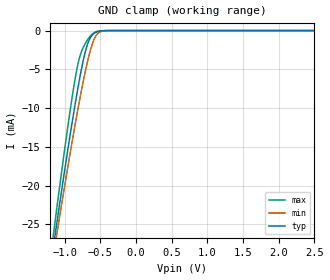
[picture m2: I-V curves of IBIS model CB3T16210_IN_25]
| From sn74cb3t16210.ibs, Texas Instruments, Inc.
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[Model]   CB3T16210_IN_25
Model_type  Input
Vinl=0.7
Vinh=1.7
| variable   typ   min   max
C_comp   2.65pF   2.04pF   3.27pF
[Temperature Range]   40   100   -40
| Ambient temperature   25   85   -40
[Voltage range]   2.5   2.3   2.7
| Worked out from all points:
|   GND clamp passes 1 mA (typ) near -0.64 V on its own axis
[GND Clamp]
| CB3T16210_IN_25
|   Voltage   I(typ)   I(min)   I(max)
-5.5V     -338.9mA   -314.3mA   -369mA
-1.17V    -28.73mA   -29.82mA   -27.27mA
-1.13V    -26.19mA   -27.5mA    -24.42mA
-1.095V   -23.98mA   -25.48mA   -21.95mA
-925mV    -13.65mA   -15.98mA   -10.52mA
-825mV    -8.06mA    -10.74mA   -4.88mA
-775mV    -5.531mA   -8.266mA   -3.027mA
-700mV    -2.416mA   -4.874mA   -1.51mA
-590mV    -396.4uA   -1.217mA   -293.2uA
-515mV    -88.16uA   -231.8uA   -44.89uA
-395mV    -4.232uA   -9.445uA   -775nA
2.5V      57.25pA    176.8pA    32.61pA
